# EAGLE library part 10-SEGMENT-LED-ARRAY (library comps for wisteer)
DC-7G3EWA :led array (rs 247-3107) http://radiospares-fr.rs-online.com/web/p/afficheurs-led/2473107/
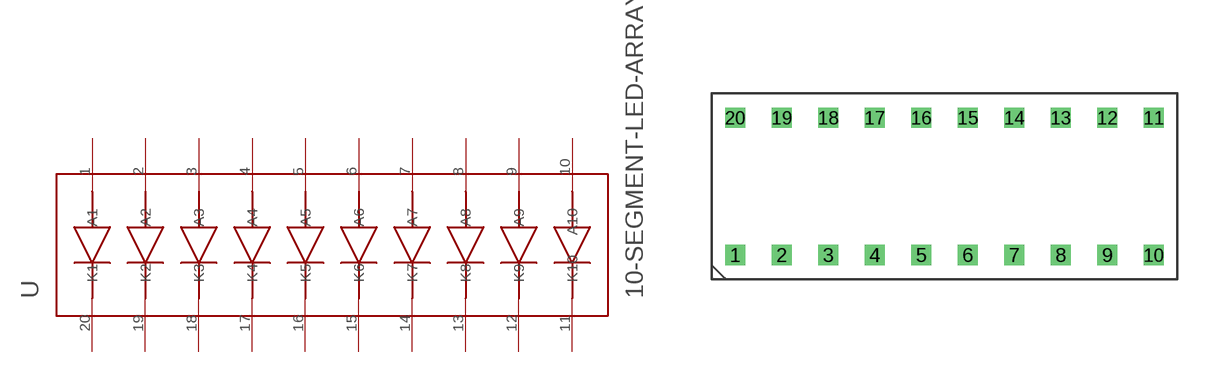
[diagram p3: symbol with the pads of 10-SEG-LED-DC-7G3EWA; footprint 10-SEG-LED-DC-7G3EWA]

Designator prefix -

## 10-SEGMENT-LED-ARRAY  [10-SEG-LED-DC-7G3EWA]
1  A1
2  A2
3  A3
4  A4
5  A5
6  A6
7  A7
8  A8
9  A9
10  A10
11  K10
12  K9
13  K8
14  K7
15  K6
16  K5
17  K4
18  K3
19  K2
20  K1

## Footprint 10-SEG-LED-DC-7G3EWA (pad centres in mm)
drill 0.6 square: 1 -11.43,-3.75; 2 -8.89,-3.75; 3 -6.35,-3.75; 4 -3.81,-3.75; 5 -1.27,-3.75; 6 1.27,-3.75; 7 3.81,-3.75; 8 6.35,-3.75; 9 8.89,-3.75; 10 11.43,-3.75; 11 11.43,3.75; 12 8.89,3.75; 13 6.35,3.75; 14 3.81,3.75; 15 1.27,3.75; 16 -1.27,3.75; 17 -3.81,3.75; 18 -6.35,3.75; 19 -8.89,3.75; 20 -11.43,3.75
